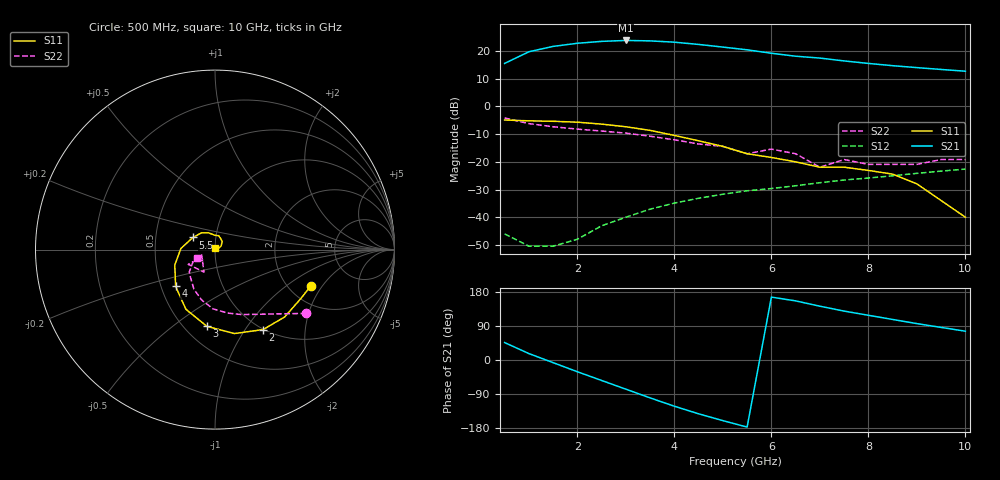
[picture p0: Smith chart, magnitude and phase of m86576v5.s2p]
!  MGA-86576 S AND NOISE PARAMETERS
!  Vd = 5 V  LAST UPDATED 06-27-94
# ghz s ma r 50
!FREQ  S11  S21  S12  S22
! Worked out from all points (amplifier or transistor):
!   20 points, 500 MHz to 10 GHz, reference 50 ohm
!   highest |S21| = 23.8 dB at 3 GHz (marker M1)
!   |S21| within 3 dB of that: 1.28 GHz to 5.307 GHz (4.027 GHz wide, 122 % of centre)
!   unconditionally stable (mu >= 1): start of sweep to end of sweep
!   at 2 GHz: K = 5.82, MAG = 24.8 dB, |S12| = -48.0 dB
!   at 5.5 GHz: K = 1.68, MAG = 20.6 dB, |S12| = -30.5 dB
!   at 10 GHz: K = 1.70, MAG = 12.8 dB, |S12| = -22.6 dB
!   lowest NFmin = 1.50 dB at 2.5 GHz
!   S11 on the Smith chart (normalised r, x): 500 MHz: 2.59, -1.57; 2 GHz: 0.99, -1.21; 3 GHz: 0.64, -0.67; 4 GHz: 0.60, -0.27; 5.5 GHz: 0.78, +0.11; 10 GHz: 1.00, +0.02
0.5  0.57 -21.0  5.99 46.0  0.005 -15.0  0.62 -35.0
1  0.55 -30.0  9.72 17.0  0.003 11.0  0.49 -47.0
1.5  0.54 -44.0  12.15 -7.0  0.003 58.0  0.43 -57.0
2  0.52 -59.0  13.84 -31.0  0.004 85.0  0.39 -68.0
2.5  0.48 -77.0  14.98 -54.0  0.007 96.0  0.36 -79.0
3  0.43 -96.0  15.56 -77.0  0.01 100.0  0.33 -92.0
3.5  0.37 -116.0  15.28 -100.0  0.014 99.0  0.29 -105.0
4  0.3 -137.0  14.49 -122.0  0.018 95.0  0.25 -118.0
4.5  0.24 -159.0  13.18 -142.0  0.022 92.0  0.21 -130.0
5  0.19 178.0  11.82 -160.0  0.026 89.0  0.19 -139.0
5.5  0.14 151.0  10.54 -177.0  0.03 85.0  0.14 -151.0
6  0.12 129.0  9.14 166.0  0.033 81.0  0.17 -151.0
6.5  0.1 111.0  8.08 156.0  0.037 82.0  0.14 -116.0
7  0.08 91.0  7.48 142.0  0.042 76.0  0.08 -158.0
7.5  0.08 75.0  6.64 129.0  0.047 72.0  0.11 -153.0
8  0.07 64.0  5.99 118.0  0.051 69.0  0.09 -151.0
8.5  0.06 48.0  5.45 107.0  0.056 65.0  0.09 -146.0
9  0.04 31.0  5.03 96.0  0.062 62.0  0.09 -140.0
9.5  0.02 18.0  4.66 86.0  0.068 58.0  0.11 -143.0
10  0.01 93.0  4.33 76.0  0.074 53.0  0.11 -154.0
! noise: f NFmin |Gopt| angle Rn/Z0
1  2.1  0.56  27  0.43
1.5  1.6  0.54  31  0.4
2.5  1.5  0.47  40  0.36
4  1.6  0.38  54  0.32
6  1.8  0.28  77  0.28
8  2.1  0.22  107  0.25
